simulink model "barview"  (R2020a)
settings: Solver=FixedStepDiscrete  StartTime=0.0  StopTime=15  FixedStep=0.001  RelTol=1e-3  EnableMultiTasking=on

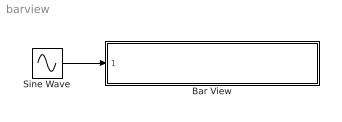
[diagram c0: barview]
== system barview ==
  Bar View : Subsystem  mask(Bar View){max=100, limit=80, color_ok=[0.0, 1.0, 0.0], color_max=[1.0, 0.0, 0.0]}
      mask prompts: max "Maximalwert"; limit "Grenzwert"; color_ok "Farbe fuer normale Werte"; color_max "Farbe fuer grosse Werte"
      mask help: Zeigt ein (positives) Signal als Farbbalken an.
  Sine Wave : Sin  Amplitude=60  Bias=50  SampleTime=0
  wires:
  Sine Wave/1 -> Bar View/1(In)

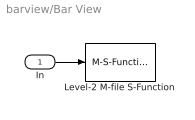
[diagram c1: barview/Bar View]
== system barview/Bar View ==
  In : Inport
  Level-2 M-file S-Function : M-S-Function  FunctionName=sfun_barview  Parameters=max,limit,color_ok,color_max
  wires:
  In/1 -> Level-2 M-file S-Function/1
